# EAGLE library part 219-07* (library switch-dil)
Surface Mount DIP Switch Series 219 SMT CTS Electronic Components Sourc: www.ctscorp.com
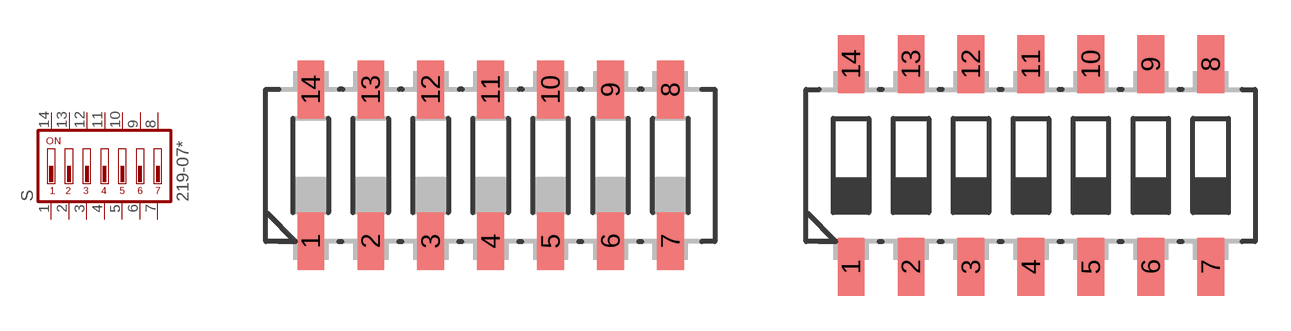
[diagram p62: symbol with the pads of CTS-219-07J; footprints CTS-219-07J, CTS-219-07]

Designator prefix S

## 219-07J (OC_FARNELL: unknown; OC_NEWARK: unknown)  [CTS-219-07J]
1  1  pas
2  2  pas
3  3  pas
4  4  pas
5  5  pas
6  6  pas
7  7  pas
8  8  pas
9  9  pas
10  10  pas
11  11  pas
12  12  pas
13  13  pas
14  14  pas

## 219-07 (OC_FARNELL: unknown; OC_NEWARK: unknown)  [CTS-219-07]
Pads as for CTS-219-07J

## Footprint CTS-219-07J (pad centres in mm)
Surface Mount DIP Switch Series 219 SMT "J" Bend CTS Electronic Components Sourc: www.ctscorp.com
smd 1.13 x 2.44: 1 -7.62,-3.215; 2 -5.08,-3.215; 3 -2.54,-3.215; 4 0,-3.215; 5 2.54,-3.215; 6 5.08,-3.215; 7 7.62,-3.215; 8 7.62,3.215; 9 5.08,3.215; 10 2.54,3.215; 11 0,3.215; 12 -2.54,3.215; 13 -5.08,3.215; 14 -7.62,3.215

## Footprint CTS-219-07 (pad centres in mm)
Surface Mount DIP Switch Series 219 SMT CTS Electronic Components Sourc: www.ctscorp.com
smd 1.13 x 2.44: 1 -7.62,-4.3; 2 -5.08,-4.3; 3 -2.54,-4.3; 4 0,-4.3; 5 2.54,-4.3; 6 5.08,-4.3; 7 7.62,-4.3; 8 7.62,4.3; 9 5.08,4.3; 10 2.54,4.3; 11 0,4.3; 12 -2.54,4.3; 13 -5.08,4.3; 14 -7.62,4.3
